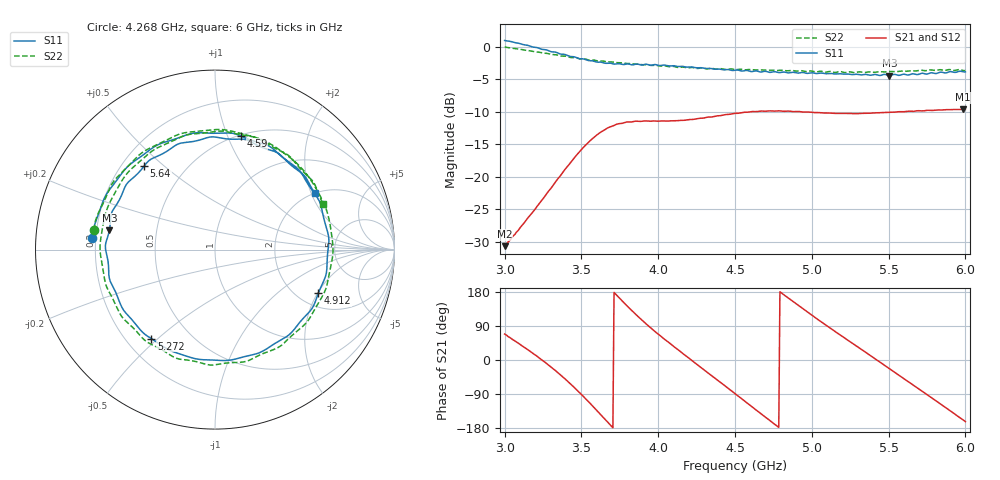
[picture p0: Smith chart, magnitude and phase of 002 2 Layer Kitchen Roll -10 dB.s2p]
!  04/11/2025  13:43:37
! Ref Plane: 0.000 mm
# MHZ S MA R  50
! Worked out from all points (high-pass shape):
!   401 points, 3 GHz to 6 GHz, reference 50 ohm
!   highest |S21| = -9.64 dB at 5.985 GHz (marker M1); lowest = -30.7 dB at 3 GHz (marker M2)
!   |S21| within 3 dB of the highest: 3.661 GHz to end of sweep
!   lowest |S11| = -4.5 dB at 5.505 GHz (marker M3), VSWR 3.98, Z = 12.7 + j4.25 ohm
!   |S11| at or under -10 dB: nowhere
!   |S22| runs from -4.0 to -0.1 dB; largest |S21 - S12| = 0.0077
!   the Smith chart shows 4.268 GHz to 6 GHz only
!   S11 on the Smith chart (normalised r, x): 4.268 GHz: 0.19, +0.04; 4.59 GHz: 0.51, +1.12; 4.912 GHz: 2.55, -2.03; 5.272 GHz: 0.30, -0.48; 5.64 GHz: 0.29, +0.43; 6 GHz: 2.00, +2.12
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3000  1.114 -114.2  0.02923 68.5  0.02944 69.6  0.9932 -116.6
3142.5  1.026 -148.2  0.04659 29.7  0.0467 30.6  0.935 -150.2
3270  0.9443 178.5  0.07311 -8.1  0.07305 -7.0  0.8879 175.2
3390  0.8705 141.4  0.1125 -48.6  0.1129 -47.8  0.8447 136.5
3502.5  0.8056 99.8  0.1626 -92.0  0.1628 -91.4  0.8035 93.8
3637.5  0.7541 42.2  0.2237 -149.5  0.2252 -148.8  0.7742 37.1
3735  0.7378 -1.7  0.2541 168.5  0.2548 169.7  0.7514 -4.6
3862.5  0.7336 -54.2  0.2668 117.0  0.2686 118.4  0.7326 -55.6
4005  0.7157 -104.1  0.2671 66.8  0.2667 67.9  0.7098 -105.1
4147.5  0.7047 -149.1  0.2708 21.2  0.2728 22.0  0.6948 -151.1
4267.5  0.6873 174.7  0.2807 -16.6  0.2825 -15.6  0.6814 170.9
4500  0.6579 104.3  0.3067 -88.8  0.3085 -88.0  0.6658 97.1
4590  0.6496 77.3  0.314 -116.8  0.3159 -116.0  0.666 67.8
4755  0.641 25.0  0.319 -168.6  0.3203 -167.7  0.6575 15.2
4912.5  0.6249 -22.9  0.3168 143.8  0.3176 144.8  0.6487 -32.9
5002.5  0.6288 -49.1  0.3116 117.6  0.3123 118.5  0.6474 -58.6
5272.5  0.6094 -125.5  0.3052 41.7  0.3066 42.4  0.631 -134.4
5505  0.5981 169.6  0.3126 -22.4  0.3145 -21.6  0.6422 161.2
5640  0.6098 130.5  0.3183 -60.4  0.3204 -59.5  0.6509 123.1
5820  0.6254 79.4  0.3258 -111.2  0.3277 -110.3  0.6611 72.9
5985  0.6398 34.4  0.3295 -158.0  0.3316 -157.1  0.6543 27.6
6000  0.6385 29.5  0.329 -162.6  0.3306 -161.7  0.6539 22.7
